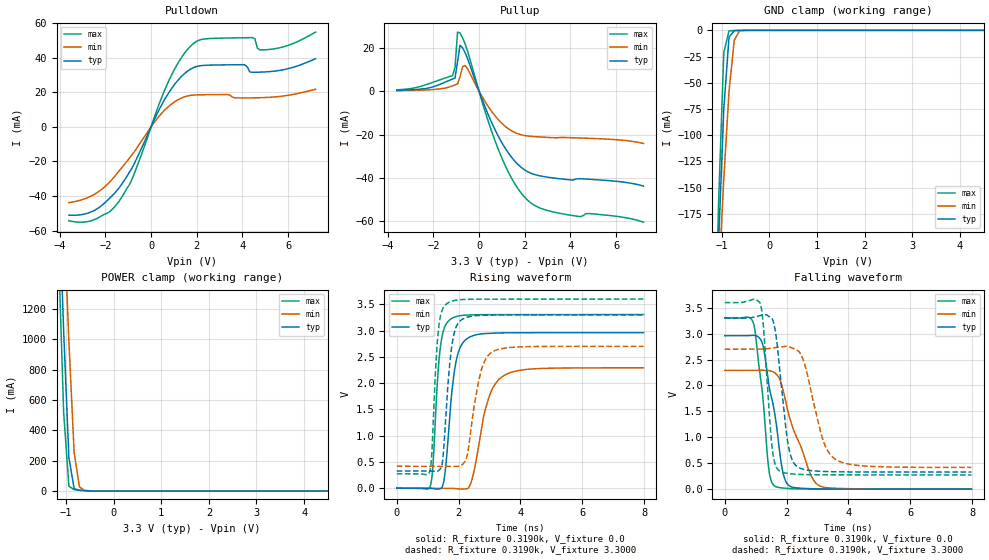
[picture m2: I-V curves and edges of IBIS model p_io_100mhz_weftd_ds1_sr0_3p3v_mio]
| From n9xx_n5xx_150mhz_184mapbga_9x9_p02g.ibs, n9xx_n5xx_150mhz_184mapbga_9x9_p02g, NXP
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[Model] p_io_100mhz_weftd_ds1_sr0_3p3v_mio
|   Model p_io_100mhz_weftd_ds1_sr0_3p3v_mio
| This model was characterised for following simulation conditions:
| External (pad) voltage:
|   - Typ: 3.3V,   - Min: 2.7V,   - Max: 3.6V
| Library cells for typ/min/max conditions are connected as defined below:
|  pad - External Pad
|  ipp_do_lv - Core Input
|  ipp_obe_lv - Output Buffer Enable
|  IOGC - NC
|  REFH3V3 - REFH3V3
|  REFL3V3 - REFL3V3
|  ZI - NC
|  abut_ncal_vddio[1] - vddio
|  abut_ncal_vddio[2] - vddio
|  abut_ncal_vddio[3] - vssio
|  abut_ncal_vddio[4] - vddio
|  abut_ncal_vddio[5] - vddio
|  abut_ncal_vddio[6] - vssio
|  abut_pcal_vddio[1] - vssio
|  abut_pcal_vddio[2] - vssio
|  abut_pcal_vddio[3] - vddio
|  abut_pcal_vddio[4] - vssio
|  abut_pcal_vddio[5] - vssio
|  abut_pcal_vddio[6] - vddio
|  ipp_do_1p8v - ipp_do_1p8v
|  ipp_dse_lv - vdd_lv
|  ipp_eftd_lv - NC
|  ipp_ina_mux_vddio - NC
|  ipp_ina_mux_vddio[0] - NC
|  ipp_ina_mux_vddio[1] - NC
|  ipp_ina_r0_vddio - NC
|  ipp_ina_r0a_vddio - NC
|  ipp_ina_r0b_vddio - NC
|  ipp_ina_r0c_vddio - NC
|  ipp_ina_r0d_vddio - NC
|  ipp_ina_r0e_vddio - NC
|  ipp_ina_r0f_vddio - NC
|  ipp_ina_r300_vddio - NC
|  ipp_ina_r300a_vddio - NC
|  ipp_ina_r300b_vddio - NC
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Model_type I/O
Polarity   Non-Inverting
Enable   Active-High
Vinl =   0.9900V
Vinh =   2.3100V
Vmeas =  1.6500V
Cref =   30.0000pF
Rref =   1.0000M
Vref =   3.3000V
C_comp   1.3824pF   1.3233pF   1.4661pF
|C_comp_pullup   0.6933pF   0.7248pF   0.6716pF
|C_comp_pulldown   0.6080pF   0.6608pF   0.5695pF
[Model Spec]
| variable   typ   min   max
Vinh   2.3100V   1.8900V   2.5200V
Vinl   0.9900V   0.8100V   1.0800V
[Temperature Range]   25.0000   0.1250k   -40.0000
[Voltage Range]   3.3000V   2.7000V   3.6000V
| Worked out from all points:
|   slope of the pulldown table from 0 to 0.495 V, typ, clamps not added: 36.8 ohm
|   slope of the pullup table from 0 to 0.495 V, typ, clamps not added: 37.8 ohm
|   GND clamp passes 1 mA (typ) near -0.75 V on its own axis
|   POWER clamp passes 1 mA (typ) near -0.55 V on its own axis
|   rising waveform, R_fixture 0.3190k, V_fixture 0.0: 20-80 % time 291ps typ, 502ps min, 208ps max; typ from 0 V to 2.96 V
|   rising waveform, R_fixture 0.3190k, V_fixture 3.3000: 20-80 % time 241ps typ, 386ps min, 177ps max; typ from 0.33 V to 3.3 V
|   falling waveform, R_fixture 0.3190k, V_fixture 0.0: 20-80 % time 457ps typ, 746ps min, 320ps max; typ from 2.96 V to 0 V
|   falling waveform, R_fixture 0.3190k, V_fixture 3.3000: 20-80 % time 322ps typ, 564ps min, 230ps max; typ from 3.3 V to 0.33 V
[Pulldown]
|Voltage   I(typ)   I(min)   I(max)
-3.6V     -50.99mA   -43.76mA   -54.26mA
-2.5V     -48.39mA   -39.11mA   -53.69mA
-1.4V     -35.22mA   -25.46mA   -42.92mA
-850mV    -24.19mA   -16.4mA    -30.7mA
800mV     20.23mA    12.14mA    27.32mA
1.35V     29.37mA    16.76mA    40.44mA
1.9V      34.45mA    18.38mA    48.57mA
4.1V      35.83mA    16.68mA    51.45mA
4.43V     31.54mA    16.72mA    51.52mA
4.65V     31.54mA    16.77mA    45.56mA
5.09V     31.78mA    16.98mA    44.58mA
7.2V      39.32mA    21.7mA     54.71mA
[Pullup]
|Voltage   I(typ)   I(min)   I(max)
-3.6V     392.3uA    235.2uA    607.2uA
-1.16V    5.571mA    2.41mA     7.094mA
-1.05V    6.017mA    2.857mA    10.99mA
-940mV    13.55mA    3.321mA    27.21mA
-830mV    21.12mA    6.673mA    26.77mA
-720mV    20.02mA    11.25mA    24.57mA
-610mV    17.72mA    11.8mA     21.82mA
820mV     -20.27mA   -12.85mA   -26.19mA
1.48V     -31.2mA    -18.62mA   -41.17mA
2.03V     -36.53mA   -20.52mA   -49.25mA
3.46V     -40.29mA   -21.47mA   -56.15mA
7.2V      -43.77mA   -24.12mA   -60.4mA
[GND_clamp]
|Voltage   I(typ)   I(min)   I(max)
-3.6V     -4.179A    -3.084A    -5.65A
-1.18V    -350.3mA   -344.8mA   -366.5mA
-1.07V    -203.5mA   -240.3mA   -165.6mA
-960mV    -75.17mA   -142.1mA   -21.27mA
-850mV    -6.53mA    -58.02mA   -538.4uA
-740mV    -289.9uA   -9.332mA   -209.1uA
-630mV    -85.04uA   -601.4uA   -92.54uA
-300mV    -199.1nA   -1.25uA    -48.79nA
7.2V      0A         0A         0A
[POWER_clamp]
|Voltage   I(typ)   I(min)   I(max)
-3.6V     24.55A     22.33A     26.93A
-1.16V    2.047A     2.721A     1.599A
-1.05V    1.052A     1.848A     514.6mA
-940mV    218.8mA    982.2mA    31.26mA
-830mV    15.16mA    252.6mA    8.517mA
-720mV    4.307mA    26.88mA    4.483mA
-610mV    1.728mA    3.641mA    1.672mA
7.2V      0A         0A         0A
[Ramp]
| variable   typ   min   max
dV/dt_r  1.7760/0.2909n   1.3748/0.5021n   1.9829/0.2081n
dV/dt_f  1.7821/0.3218n   1.3685/0.5644n   1.9953/0.2303n
R_load = 0.3190k
[Rising Waveform]
R_fixture= 0.3190k
V_fixture= 0.0
V_fixture_min= 0.0
V_fixture_max= 0.0
|time   V(typ)   V(min)   V(max)
0s        3.011nV    251.5nV    9.8nV
1.08ns    -142.9uV   -133.7uV   31.55mV
1.404ns   -9.73mV    470.1uV    2.659V
1.556ns   269.7mV    1.193mV    3.079V
1.749ns   1.634V     -839.2uV   3.221V
2.162ns   2.787V     -14.31mV   3.292V
2.435ns   2.897V     171.7mV    3.3V
2.995ns   2.95V      1.754V     3.304V
3.482ns   2.957V     2.15V      3.304V
7.98ns    2.96V      2.291V     3.305V
[Rising Waveform]
R_fixture= 0.3190k
V_fixture= 3.3000
V_fixture_min= 2.7000
V_fixture_max= 3.6000
|time   V(typ)   V(min)   V(max)
0s        329.6mV    418.3mV    274.4mV
1.068ns   329.7mV    418.1mV    321.5mV
1.345ns   331.7mV    418.4mV    3.001V
1.486ns   541.5mV    419.1mV    3.417V
1.618ns   1.677V     418.8mV    3.512V
1.957ns   3.115V     416.5mV    3.582V
2.259ns   3.251V     582.6mV    3.595V
2.688ns   3.29V      2.141V     3.599V
3.086ns   3.297V     2.593V     3.599V
7.98ns    3.3V       2.7V       3.6V
[Falling Waveform]
R_fixture= 0.3190k
V_fixture= 0.0
V_fixture_min= 0.0
V_fixture_max= 0.0
|time   V(typ)   V(min)   V(max)
0s        2.96V      2.291V     3.305V
935.6ps   2.967V     2.29V      3.192V
1.225ns   2.799V     2.293V     1.822V
1.421ns   2.042V     2.288V     407.2mV
1.613ns   1.48V      2.246V     61.64mV
1.841ns   452.7mV    2.021V     24.41mV
1.995ns   128.7mV    1.632V     15.78mV
2.745ns   9.96mV     328.6mV    2.307mV
3.035ns   5.482mV    75.2mV     1.217mV
7.98ns    94.6uV     222.3uV    59.15uV
[Falling Waveform]
R_fixture= 0.3190k
V_fixture= 3.3000
V_fixture_min= 2.7000
V_fixture_max= 3.6000
|time   V(typ)   V(min)   V(max)
0s        3.3V       2.7V       3.6V
1.156ns   3.349V     2.7V       3.575V
1.258ns   3.363V     2.704V     3.1V
1.531ns   3.287V     2.723V     814.1mV
1.768ns   2.378V     2.741V     352.3mV
2.062ns   828.3mV    2.753V     301.5mV
2.399ns   414.8mV    2.656V     285.3mV
3.181ns   342.3mV    946.7mV    276.3mV
3.593ns   335.4mV    571.4mV    275.4mV
7.98ns    329.8mV    419.1mV    274.5mV
